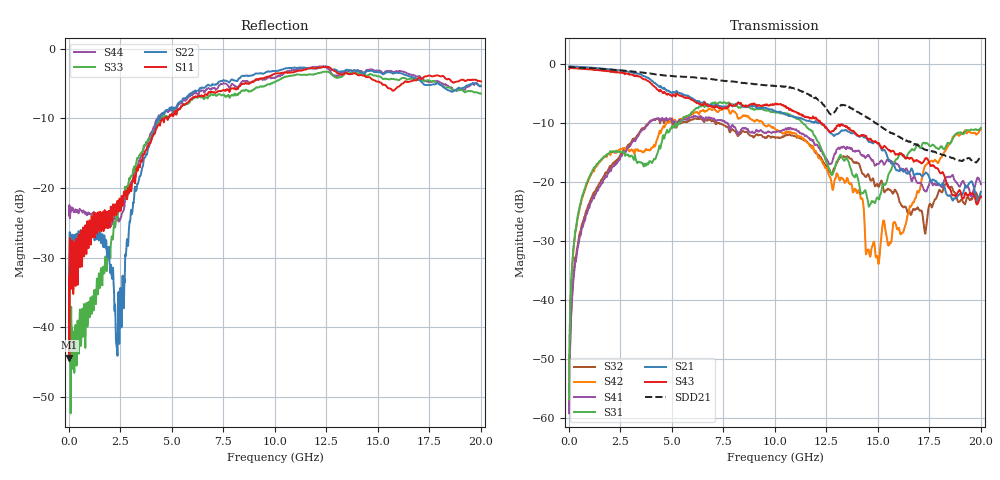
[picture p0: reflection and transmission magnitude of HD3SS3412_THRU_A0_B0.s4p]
!  4-Port S-parameters saved by WinCal
! VAR MeasName=S-Parameters (CALIBRATED_DATA) read from VNA (E8364B)
! VAR MeasDate=6/29/2011 9:41:54 AM
! VAR NAME=Measurement
! VAR FILENAME=HD3SS3412_THRU_A0_B0.s4p
! VAR DATE=6/29/2011 9:41:55 AM
! VAR PHYS_PORTS=1,2,3,4
# Hz S RI R 50
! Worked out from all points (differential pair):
!   1601 points, 10 MHz to 20.01 GHz, reference 50 ohm
!   strongest paths, dB at 10 MHz, 5.009 GHz, 10.01 GHz, 15.01 GHz, 20.01 GHz:
!     S43: -0.8, -5.4, -6.7, -13.3, -22.5
!     S21: -0.3, -4.9, -7.9, -13.4, -21.6
!     S31: -56.8, -10.5, -8.2, -22.7, -10.7
!     S41: -59.1, -9.3, -11.5, -16.9, -20.3
!     S42: -49.8, -9.1, -10.9, -33.2, -11.0
!     S32: -57.7, -9.7, -12.4, -20.6, -22.3
!   taken as a pair (ports 3,1 in; 4,2 out), SDD21 dB: -0.6, -2.0, -3.6, -10.2, -15.8
!   lowest |S11| = -44.3 dB at 22.5 MHz (marker M1), VSWR 1.01, Z = 50.6 - j0.253 ohm
!   |S11| at or under -10 dB: start of sweep to 4.65 GHz; 4.771 GHz to 4.819 GHz (48.55 MHz wide, 1.01 % of centre)
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1e7  0.00365 -0.0229  0.9657 0.0295  -0.000315 0.00111  0.00122 -0.000141
     0.9619 -0.014  0.0196 0.00599  -0.000675 -0.000223  0.00112 0.000936
     0.00122 0.00078  1.81e-05 -0.0013  -0.0145 -0.02  0.9841 0.0482
     0.000458 -0.001  0.00143 0.00291  0.9113 -0.0544  0.0535 0.0342
2.24975e7  0.00552 -0.0025  0.9637 -0.00501  0.000336 0.00287  -8.8e-05 -0.00187
           0.9647 -0.0146  0.0336 0.00721  -2.43e-05 -0.00203  0.000458 0.00278
           0.000128 0.00309  -0.000265 -0.00173  -0.0213 0.0173  0.9879 0.00682
           -0.000308 -0.00186  0.00038 0.00267  0.9242 -0.0308  0.0749 -0.00912
9.34815e8  0.0367 0.0173  0.8384 -0.4186  0.0479 0.0917  -0.0299 -0.0533
           0.8561 -0.3929  0.0375 0.0157  -0.0292 -0.0545  0.0447 0.0958
           0.0467 0.0964  -0.0301 -0.0564  0.0135 -0.00253  0.8707 -0.4089
           -0.0261 -0.0535  0.0408 0.0945  0.8345 -0.3618  0.0631 -0.0213
2.372028e9  0.0307 -0.071  0.3579 -0.8093  0.1566 0.0799  -0.1403 -0.0557
            0.4222 -0.7869  0.00148 0.00784  -0.1416 -0.0597  0.1515 0.1115
            0.1562 0.0953  -0.1454 -0.0618  -0.0339 -0.0537  0.4107 -0.8094
            -0.1287 -0.0752  0.1388 0.1193  0.4457 -0.7321  -0.0279 -0.0553
4.021698e9  -0.2254 0.0222  -0.3323 -0.6398  0.1127 0.0839  -0.2666 0.2055
            -0.2451 -0.6864  -0.13 0.1856  -0.2662 0.1865  0.161 0.1205
            0.1048 0.1035  -0.2765 0.1929  -0.2223 0.0837  -0.2689 -0.6709
            -0.3095 0.1225  0.139 0.1393  -0.1622 -0.6645  -0.2179 0.1217
1.49945e10  0.4244 -0.3926  0.1784 0.0349  -0.0377 0.0473  -0.0828 -0.0779
            0.1818 0.1114  0.4812 -0.4768  -0.0594 -0.0689  -0.019 0.00997
            -0.0659 0.0334  -0.0564 -0.0758  0.5217 -0.3581  0.177 0.1104
            -0.00236 -0.1435  -0.0231 0.000873  0.1296 0.1732  0.5782 -0.3804
2.0006e10  0.1029 -0.5726  0.0555 -0.0308  0.2056 0.00649  -0.0369 0.055
           0.0827 0.0103  0.0882 -0.5306  -0.0648 -0.0295  0.2109 0.1402
           0.2222 0.1877  -0.0686 -0.0342  0.1448 -0.4539  0.0595 -0.0413
           -0.0911 -0.0325  0.0823 0.2701  0.075 0.0033  0.1552 -0.5184
